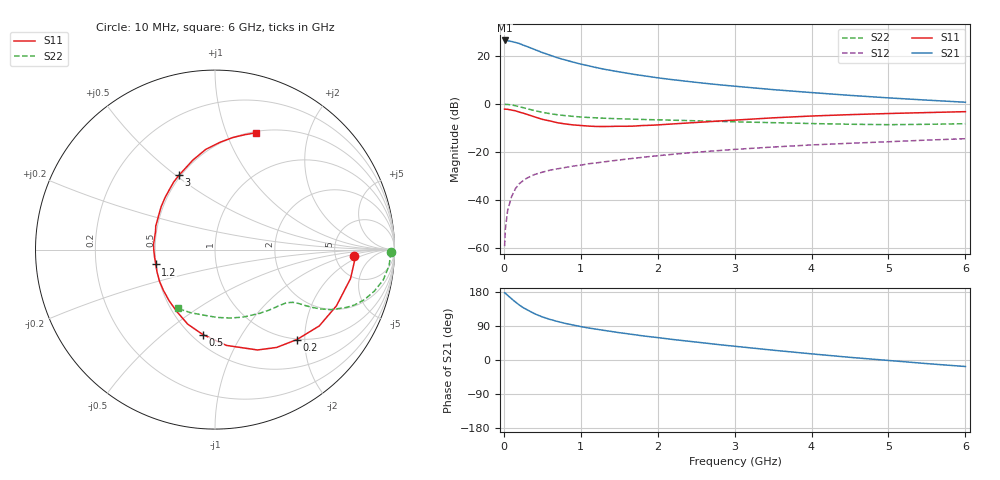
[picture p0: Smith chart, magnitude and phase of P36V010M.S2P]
! SIEMENS Small Signal Semiconductors
! BFP181
! Si NPN RF Bipolar Junction Transistor in SOT143
! VCE = 6 V  IC = 10 mA
! Common Emitter S-Parameters:  March  1996
# GHz  S  MA  R  50
!  f  S11  S21  S12  S22
! GHz  MAG  ANG  MAG  ANG  MAG  ANG  MAG  ANG
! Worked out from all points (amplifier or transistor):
!   36 points, 10 MHz to 6 GHz, reference 50 ohm
!   highest |S21| = 26.4 dB at 10 MHz (marker M1)
!   |S21| within 3 dB of that: start of sweep to 339.5 MHz
!   unconditionally stable (mu >= 1): 1.27 GHz to end of sweep
!   at 250 MHz: K = 0.31, MSG = 28.2 dB, |S12| = -31.9 dB
!   at 1.4 GHz: K = 1.03, MAG = 17.7 dB, |S12| = -23.7 dB
!   at 6 GHz: K = 1.02, MAG = 6.7 dB, |S12| = -14.5 dB
!   S11 on the Smith chart (normalised r, x): 10 MHz: 7.74, -1.44; 200 MHz: 0.99, -1.83; 500 MHz: 0.57, -0.69; 1.2 GHz: 0.50, -0.09; 3 GHz: 0.49, +0.51; 6 GHz: 0.51, +1.28
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0.01  0.778 -2.7  20.91 177.4  0.0011 82.1  0.9817 -0.8
0.02  0.7794 -5.0  20.74 176.2  0.0025 87.6  0.9776 -2.0
0.05  0.7721 -12.1  20.61 170.5  0.0062 88.6  0.9742 -5.2
0.1  0.7458 -24.8  19.91 161.7  0.0117 77.7  0.9525 -10.2
0.15  0.72 -36.2  19.01 153.1  0.0172 72.1  0.9185 -14.5
0.2  0.6778 -47.7  18.07 145.3  0.0219 67.5  0.8792 -18.4
0.25  0.6442 -57.8  16.78 138.4  0.0253 64.0  0.8373 -21.6
0.3  0.6075 -67.0  15.67 132.8  0.0287 60.3  0.7971 -23.9
0.4  0.538 -83.1  13.57 122.0  0.0341 56.6  0.727 -27.4
0.5  0.4784 -98.1  11.73 113.7  0.038 52.4  0.6704 -29.5
0.6  0.4424 -110.1  10.34 107.1  0.0419 50.9  0.6271 -30.8
0.7  0.4056 -121.6  9.086 101.6  0.0448 49.8  0.5951 -31.7
0.9  0.3663 -141.8  7.42 92.3  0.0509 48.7  0.5513 -32.9
1.1  0.3463 -158.8  6.212 84.5  0.057 48.8  0.523 -34.2
1.2  0.3399 -165.9  5.715 81.4  0.0593 48.4  0.5137 -35.0
1.7  0.3465 162.9  4.105 66.7  0.0745 47.5  0.481 -39.7
2.2  0.384 141.3  3.188 54.1  0.0897 45.4  0.4589 -45.9
3  0.4605 115.8  2.339 36.3  0.1133 40.4  0.4247 -58.1
3.5  0.5136 103.9  1.985 25.9  0.127 36.8  0.4078 -67.2
4.5  0.5987 87.3  1.507 7.0  0.152 29.1  0.3779 -88.4
5.5  0.6611 75.5  1.2 -9.5  0.1769 22.0  0.3767 -110.8
6  0.6907 70.5  1.085 -17.2  0.189 18.0  0.3879 -122.3
